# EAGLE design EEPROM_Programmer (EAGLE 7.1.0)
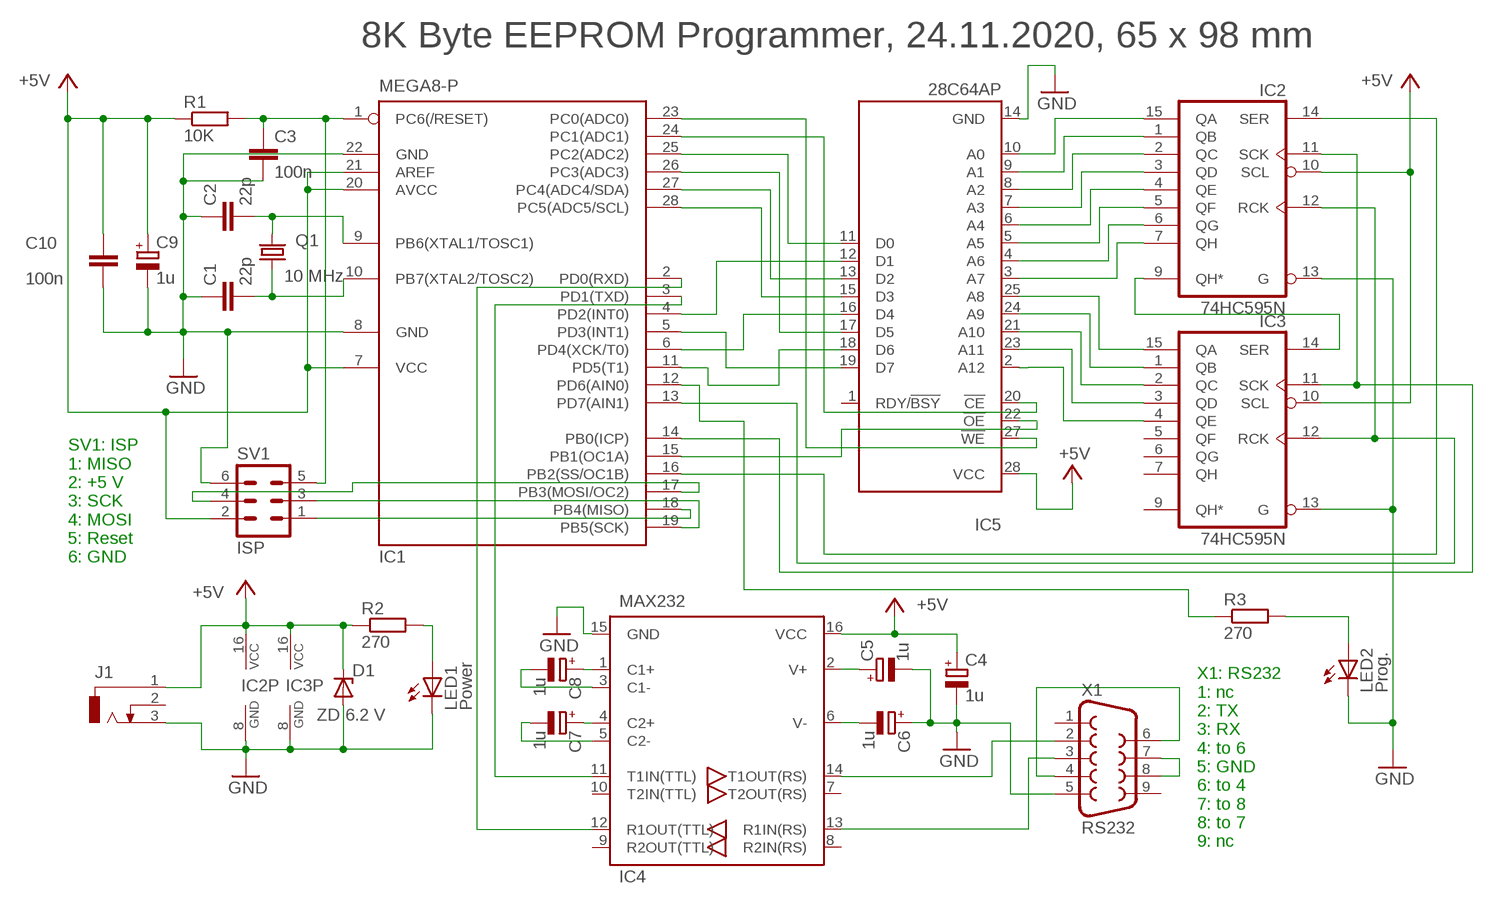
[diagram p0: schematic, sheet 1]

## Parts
C1  22p  C-EUC1206  [C1206]
C2  22p  C-EUC1206  [C1206]
C3  100n  C-EUC1206  [C1206]
C4  1u  CPOL-EUE2.5-5  [E2,5-5]
C5  1u  CPOL-EUE2.5-5  [E2,5-5]
C6  1u  CPOL-EUE2.5-5  [E2,5-5]
C7  1u  CPOL-EUE2.5-5  [E2,5-5]
C8  1u  CPOL-EUE2.5-5  [E2,5-5]
C9  1u  CPOL-EUE2.5-5  [E2,5-5]
C10  100n  C-EUC1206  [C1206]
D1  ZD 6.2 V  ZPD  [DO35Z10]
IC1  MEGA8-P  [DIL28-3]
IC2  74HC595N  [DIL16]
IC3  74HC595N  [DIL16]
IC4  MAX232-1  [DIL16]
IC5  28C64AP  [DIL28-6]
J1  DCJ0303  [DCJ0303]
LED1  Power  LED3MM  [LED3MM]
LED2  Prog.  LED3MM  [LED3MM]
Q1  10 MHz  CRYTALHC18U-V  [HC18U-V]
R1  10K  R-EU_R1206  [R1206]
R2  270  R-EU_R1206  [R1206]
R3  270  R-EU_R1206  [R1206]
SV1  ISP  ML6  [ML6]
X1  RS232  F09HP  [F09HP]

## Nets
+5V: C4.+ C9.+ C10.1 D1.C IC1.7(VCC) IC1.20(AVCC) IC1.21(AREF) IC2.10(SCL) IC2.16(VCC) IC3.10(SCL) IC3.16(VCC) IC4.16(VCC) IC5.28(VCC) J1.1 R1.1 R2.1 SV1.2
GND: C1.1 C2.1 C3.2 C4.- C5.- C6.+ C9.- C10.2 D1.A IC1.8(GND) IC1.22(GND) IC2.8(GND) IC2.13(G) IC3.8(GND) IC3.13(G) IC4.15(GND) IC5.14(GND) J1.3 LED1.K(C) LED2.K(C) SV1.6 X1.5
N$1: IC2.15(QA) IC5.10(A0)
N$2: IC2.1(QB) IC5.9(A1)
N$3: IC2.2(QC) IC5.8(A2)
N$4: IC2.3(QD) IC5.7(A3)
N$5: IC2.4(QE) IC5.6(A4)
N$6: IC2.5(QF) IC5.5(A5)
N$7: IC2.6(QG) IC5.4(A6)
N$8: IC2.7(QH) IC5.3(A7)
N$9: IC3.15(QA) IC5.25(A8)
N$10: IC3.1(QB) IC5.24(A9)
N$11: IC3.2(QC) IC5.21(A10)
N$12: IC3.3(QD) IC5.23(A11)
N$13: IC3.4(QE) IC5.2(A12)
N$14: IC2.9(QH*) IC3.14(SER)
N$15: IC1.14(PB0(ICP)) IC2.11(SCK) IC3.11(SCK)
N$16: IC1.13(PD7(AIN1)) IC2.12(RCK) IC3.12(RCK)
N$17: IC1.6(PD4(XCK/T0)) IC5.16(D4)
N$18: X1.7 X1.8
N$19: IC1.28(PC5(ADC5/SCL)) IC5.15(D3)
N$20: C2.2 IC1.9(PB6(XTAL1/TOSC1)) Q1.2
N$21: C1.2 IC1.10(PB7(XTAL2/TOSC2)) Q1.1
N$22: C3.1 IC1.1(PC6(/RESET)) R1.2 SV1.5
N$23: IC1.18(PB4(MISO)) SV1.1
N$24: IC1.2(PD0(RXD)) IC4.12(R1OUT(TTL))
N$25: C8.+ IC4.1(C1+)
N$26: C8.- IC4.3(C1-)
N$27: C6.- IC4.6(V-)
N$28: C7.+ IC4.4(C2+)
N$29: C7.- IC4.5(C2-)
N$30: C5.+ IC4.2(V+)
N$31: IC1.27(PC4(ADC4/SDA)) IC5.13(D2)
N$32: IC1.4(PD2(INT0)) IC5.12(D1)
N$33: IC1.26(PC3(ADC3)) IC5.17(D5)
N$34: IC1.25(PC2(ADC2)) IC5.11(D0)
N$35: IC1.5(PD3(INT1)) IC5.19(D7)
N$36: IC1.24(PC1(ADC1)) IC5.20(!CE)
N$37: IC1.23(PC0(ADC0)) IC5.27(!WE)
N$38: IC4.14(T1OUT(RS)) X1.2
N$39: IC1.19(PB5(SCK)) SV1.3
N$40: IC1.16(PB2(SS/OC1B)) IC2.14(SER)
N$41: IC1.17(PB3(MOSI/OC2)) SV1.4
N$42: IC4.13(R1IN(RS)) X1.3
N$43: IC1.11(PD5(T1)) IC5.18(D6)
N$44: IC1.3(PD1(TXD)) IC4.11(T1IN(TTL))
N$45: LED1.A R2.2
N$46: IC1.12(PD6(AIN0)) R3.1
N$47: LED2.A R3.2
N$48: IC1.15(PB1(OC1A)) IC5.22(!OE)
N$50: X1.4 X1.6
Unconnected: IC3.5(QF) IC3.6(QG) IC3.7(QH) IC3.9(QH*) IC4.7(T2OUT(RS)) IC4.8(R2IN(RS)) IC4.9(R2OUT(TTL)) IC4.10(T2IN(TTL)) IC5.1(RDY/!BSY) J1.2 X1.1 X1.9

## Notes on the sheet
- 8K Byte EEPROM Programmer, 24.11.2020, 65 x 98 mm
- SV1: ISP
  1: MISO
  2: +5 V
  3: SCK
  4: MOSI
  5: Reset
  6: GND
- X1: RS232
  1: nc
  2: TX
  3: RX
  4: to 6
  5: GND
  6: to 4
  7: to 8
  8: to 7
  9: nc

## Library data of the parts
C1-C3 C10 = rcl:C-EU: CAPACITOR, European symbol
C4-C9 = rcl:CPOL-EU: POLARIZED CAPACITOR, European symbol
D1 = diode:ZPD: Z DIODE
IC1 = atmel:MEGA8-P: MICROCONTROLLER 8 Kbytes FLASH, 1 kbytes SRAM, 512 bytes EEPROM, USART, 4-channel 10 bit ADC, 2-channel 8 bit ADC Pin compatible with Atmega48, ATMega88, ATMega168 Source: avr.lbr; OC_FARNELL: unknown; OC_NEWARK: unknown
IC2 IC3 = 74xx-eu:74*595: 8-bit SHIFT REGISTER, output latch
IC4 = 11manni:MAX232-1
IC5 = microchip:28*64A: CMOS EEPROM 64 K (8 K x 8), low voltage; MPN: AT28C64B-15PU; OC_FARNELL: 1631144; OC_NEWARK: 96K6557
J1 = con-jack:DCJ0303: DC POWER JACK Source: DCJ0303.pdf; OC_FARNELL: unknown; OC_NEWARK: unknown
LED1 LED2 = led:LED: LED
Q1 = 11manni:CRYTAL: CRYSTAL
R1-R3 = rcl:R-EU_: RESISTOR, European symbol
SV1 = con-harting-ml:ML6: HARTING; OC_FARNELL: unknown; OC_NEWARK: unknown
X1 = con-subd:F09: SUB-D; OC_FARNELL: unknown; OC_NEWARK: unknown

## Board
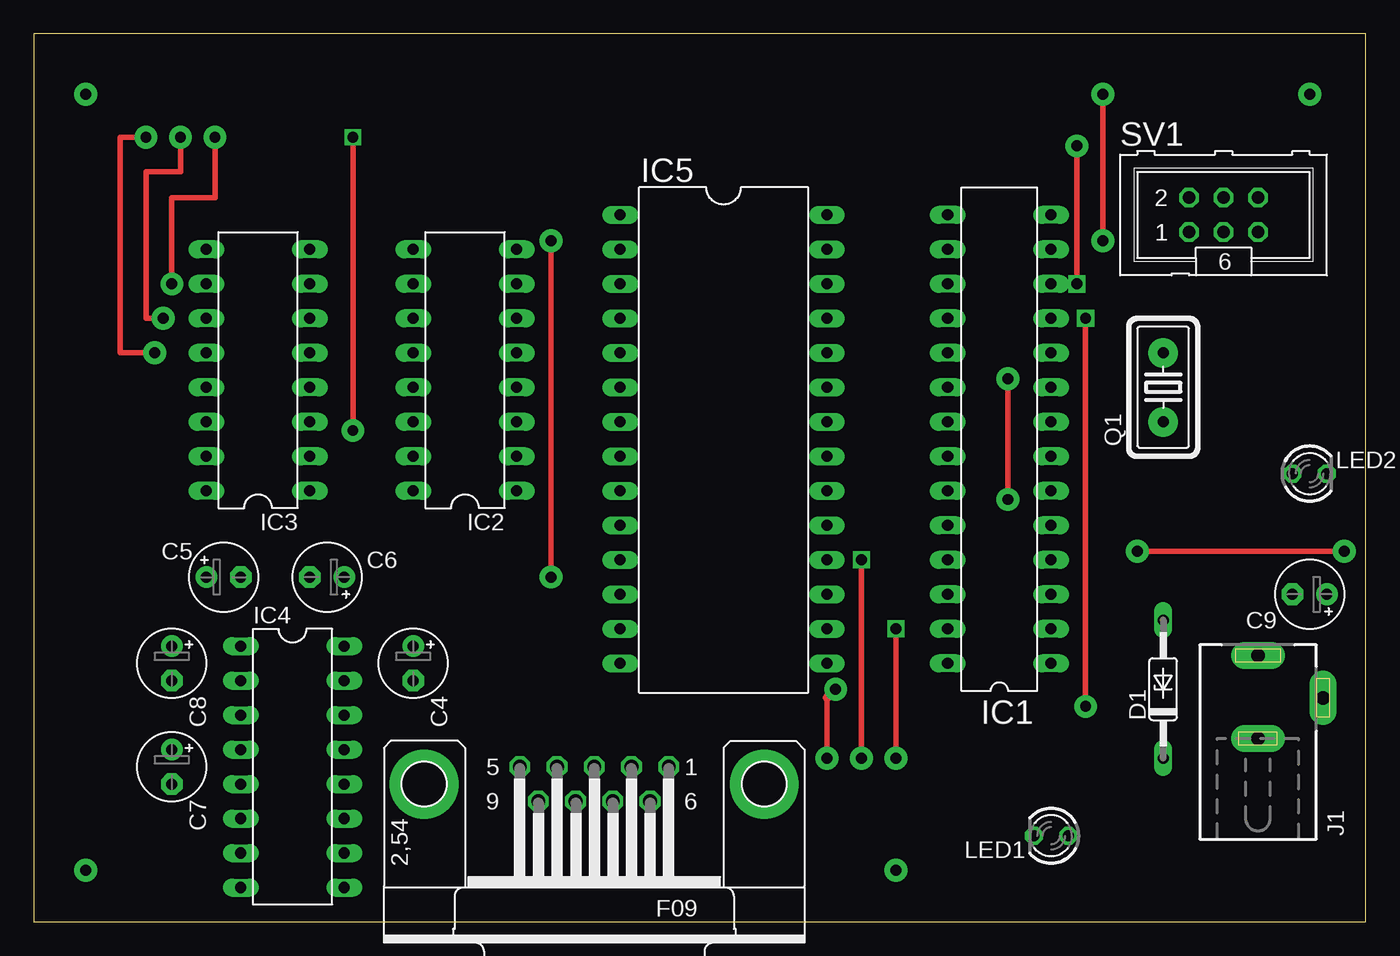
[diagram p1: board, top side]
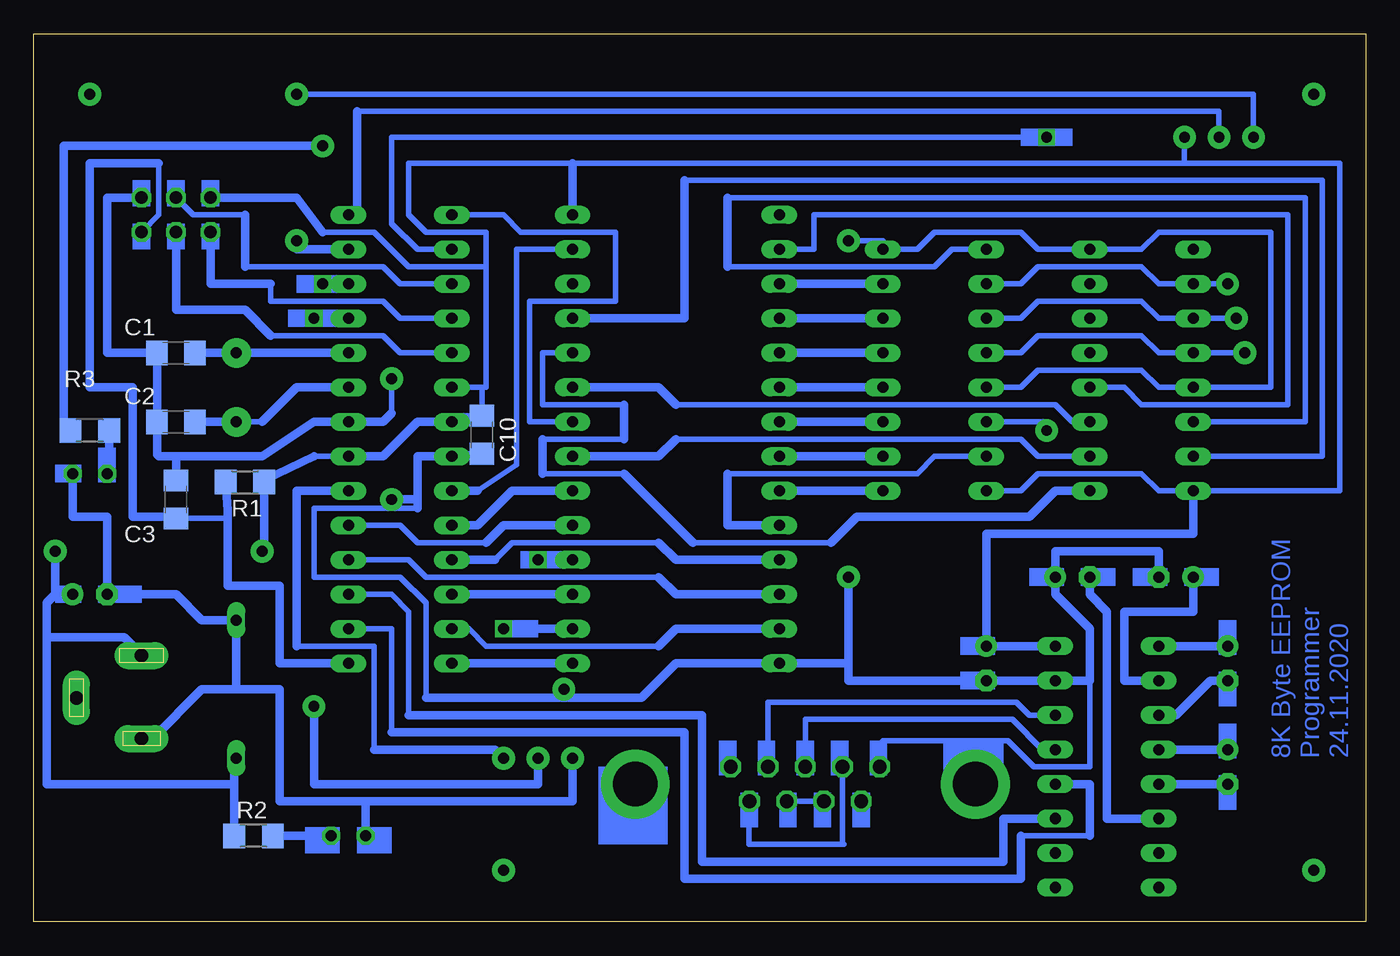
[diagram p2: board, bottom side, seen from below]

Size 98.09 x 65.39 mm. Coordinates in mm from the lower left corner, seen from the top.
Outline: 0,0 98.09,0 98.09,65.39 0,65.39 0,0
Copper layers (1*16): Top 0.035mm / dielectric 1.5mm / Bottom 0.035mm
Design rules "default": minimum track width 10mil, minimum drill 24mil, track to track 8mil, track to pad 8mil, pad to pad 8mil, via to via 8mil, smd to smd 8mil, copper to edge 40mil, drill to drill 8mil, minimum pad ring 10mil, minimum via ring 8mil, stop-mask expansion 4mil, vias tented up to drill 0mil, thermal gap 10mil

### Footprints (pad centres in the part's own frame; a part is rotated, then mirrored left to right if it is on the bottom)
C1206 = smd 1.6 x 1.8: 1 -1.4,0; 2 1.4,0
E2,5-5 = drill 0.813 pad 1.6: + -1.27,0 | drill 0.813 pad 1.6 octagon: - 1.27,0
DO35Z10 = drill 0.813 long: A 5.08,0; C -5.08,0
DIL28-3 = drill 0.813 long: 1 -16.51,-3.81; 2 -13.97,-3.81; 3 -11.43,-3.81; 4 -8.89,-3.81; 5 -6.35,-3.81; 6 -3.81,-3.81; 7 -1.27,-3.81; 8 1.27,-3.81; 9 3.81,-3.81; 10 6.35,-3.81; 11 8.89,-3.81; 12 11.43,-3.81; 13 13.97,-3.81; 14 16.51,-3.81; 15 16.51,3.81; 16 13.97,3.81; 17 11.43,3.81; 18 8.89,3.81; 19 6.35,3.81; 20 3.81,3.81; 21 1.27,3.81; 22 -1.27,3.81; 23 -3.81,3.81; 24 -6.35,3.81; 25 -8.89,3.81; 26 -11.43,3.81; 27 -13.97,3.81; 28 -16.51,3.81
DIL16 = drill 0.813 long: 1 -8.89,-3.81; 2 -6.35,-3.81; 3 -3.81,-3.81; 4 -1.27,-3.81; 5 1.27,-3.81; 6 3.81,-3.81; 7 6.35,-3.81; 8 8.89,-3.81; 9 8.89,3.81; 10 6.35,3.81; 11 3.81,3.81; 12 1.27,3.81; 13 -1.27,3.81; 14 -3.81,3.81; 15 -6.35,3.81; 16 -8.89,3.81
DIL28-6 = drill 0.813 long: 1 -16.51,-7.62; 2 -13.97,-7.62; 3 -11.43,-7.62; 4 -8.89,-7.62; 5 -6.35,-7.62; 6 -3.81,-7.62; 7 -1.27,-7.62; 8 1.27,-7.62; 9 3.81,-7.62; 10 6.35,-7.62; 11 8.89,-7.62; 12 11.43,-7.62; 13 13.97,-7.62; 14 16.51,-7.62; 15 16.51,7.62; 16 13.97,7.62; 17 11.43,7.62; 18 8.89,7.62; 19 6.35,7.62; 20 3.81,7.62; 21 1.27,7.62; 22 -1.27,7.62; 23 -3.81,7.62; 24 -6.35,7.62; 25 -8.89,7.62; 26 -11.43,7.62; 27 -13.97,7.62; 28 -16.51,7.62
DCJ0303 = drill 1 pad 2 long: 1 0,3.1; 2 4.8,0; 3 0,-3
LED3MM = drill 0.813 octagon: A -1.27,0; K 1.27,0
HC18U-V = drill 0.813 pad 2.184: 1 -2.54,0; 2 2.54,0
R1206 = smd 1.6 x 1.803: 1 -1.422,0; 2 1.422,0
ML6 = drill 0.914 octagon: 1 -2.54,-1.27; 2 -2.54,1.27; 3 0,-1.27; 4 0,1.27; 5 2.54,-1.27; 6 2.54,1.27
F09HP = drill 1.016 octagon: 1 -5.486,-1.27; 2 -2.743,-1.27; 3 0,-1.27; 4 2.743,-1.27; 5 5.486,-1.27; 6 -4.115,1.27; 7 -1.372,1.27; 8 1.372,1.27; 9 4.115,1.27 | drill 3.302 pad 5.08: G1 -12.522,0; G2 12.522,0

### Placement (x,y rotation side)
C1  87.63,41.91 0 bottom
C2  87.63,36.83 0 bottom
C3  87.63,31.11 90 bottom
C4  27.94,19.05 270 top
C5  13.97,25.4 0 top
C6  21.59,25.4 180 top
C7  10.16,11.43 270 top
C8  10.16,19.05 270 top
C9  93.98,24.13 180 top
C10  65.09,35.88 270 bottom
D1  83.19,17.14 90 top
IC1  71.12,35.56 90 top
IC2  31.75,40.64 90 top
IC3  16.51,40.64 90 top
IC4  19.05,11.43 270 top
IC5  50.8,35.56 270 top
J1  90.17,16.51 0 top
LED1  74.93,6.35 180 top
LED2  93.98,33.02 0 top
Q1  83.19,39.37 270 top
R1  82.55,32.38 180 bottom
R2  81.92,6.35 0 bottom
R3  93.98,36.2 0 bottom
SV1  87.63,52.07 0 top
X1  41.27,10.16 180 top

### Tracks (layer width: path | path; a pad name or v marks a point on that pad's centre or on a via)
+5V  (via drill 0.8 pad 1.68)
  Top 0.406: v81.28,27.3 v96.52,27.3 | v10.16,46.99 10.16,53.34 13.34,53.34 v13.34,57.78
  Bottom 0.406: IC2.16 25.4,31.75 24.13,33.02 16.51,33.02 15.24,31.75 IC3.16 1.91,31.75 1.91,55.88 13.34,55.88 | R1.1 81.13,32.54 | 77.47,34.29 IC1.7 | IC1.20 65.09,39.37 | 65.09,39.37 64.77,39.37 64.77,48.26 | 13.34,55.88 58.42,55.88 70.48,55.88 70.48,52.07 69.22,50.8 64.77,50.8 64.77,48.26 | 76.83,50.8 73.03,50.8 70.48,48.26 64.77,48.26 | 65.09,39.37 C10.1 67.31,37.28 IC1.21 | IC2.10 25.4,46.99 24.13,48.26 16.51,48.26 15.24,46.99 IC3.10 v10.16,46.99 | v13.34,57.78 13.34,55.88
  Bottom 0.61: 81.13,32.54 77.47,34.29 | IC1.7 72.39,34.29 69.85,36.83 IC1.21 | IC4.16 C4.+ 27.94,28.57 12.7,28.57 IC3.16 | IC5.28 58.42,55.88 | SV1.2 78.74,53.34 76.83,50.8 | R1.1 81.13,27.46 v81.28,27.3 | v96.52,27.3 96.52,24.13 | R2.1 83.34,10.16 | 83.34,10.16 83.34,11.91 D1.C | C9.+ 96.52,24.13 | 83.34,10.16 97.16,10.16 97.16,20.95 | 97.16,20.95 97.16,23.5 96.52,24.13 | J1.1 90.09,19.61 91.44,20.95 97.16,20.95
GND  (via drill 0.8 pad 1.68)
  Top 0.406: v38.1,25.4 v38.1,50.16 | v71.75,40.01 v71.75,31.11 | v58.42,12.06 58.42,16.51
  Top 0.61: 58.42,16.51 v59.05,17.14
  Bottom 0.406: 89.03,34.42 88.9,34.29 | 69.85,30.48 77.47,30.48 77.47,25.4 71.12,25.4 69.22,23.5 69.22,16.51 | v38.1,50.16 35.56,50.16 IC2.8 33.02,49.53 31.75,50.8 25.4,50.8 24.13,49.53 IC3.8 16.51,49.53 15.24,50.8 6.99,50.8 6.99,39.37 IC3.13 15.24,39.37 16.51,40.64 24.13,40.64 25.4,39.37 IC2.13 | 71.75,37.47 v71.75,40.01 | C10.2 67.31,34.48 IC1.22 | X1.5 35.79,13.11 35.56,13.34 26.35,13.34 24.45,11.43 20.32,11.43 20.32,17.78
  Bottom 0.61: 89.03,34.42 C2.1 C1.1 92.71,41.91 92.71,53.34 SV1.6 | 88.9,34.29 87.63,34.29 | 87.63,34.29 81.28,34.29 77.47,36.83 IC1.8 72.39,36.83 71.75,37.47 | C3.2 87.63,34.29 | IC1.22 69.85,34.29 69.85,31.11 | 69.85,31.11 69.85,30.48 | 69.22,16.51 59.05,16.51 | 59.05,16.51 53.34,16.51 50.8,19.05 IC5.14 38.1,19.05 | 38.1,19.05 v38.1,25.4 | C5.- 15.24,27.3 22.86,27.3 C6.+ 22.86,24.13 20.32,21.59 20.32,17.78 IC4.15 C4.- 38.1,17.78 38.1,19.05 | v71.75,31.11 69.85,31.11 | v59.05,17.14 59.05,16.51 | v58.42,12.06 58.42,8.89 73.66,8.89 | 73.66,8.89 80.01,8.89 80.01,17.14 83.19,17.14 | 83.19,17.14 D1.A 85.72,22.23 87.63,24.13 C9.- 92.71,29.84 95.25,29.84 LED2.K | LED1.K 73.66,8.89 | J1.3 89.36,13.51 85.72,17.14 83.19,17.14
N$1
  Bottom 0.406: IC2.15 31.75,34.29 33.02,33.02 46.99,33.02
  Bottom 0.61: 46.99,33.02 46.99,29.21 IC5.10
N$2
  Bottom 0.61: IC2.1 IC5.9
N$3
  Bottom 0.61: IC2.2 IC5.8
N$4
  Bottom 0.61: IC2.3 IC5.7
N$5
  Bottom 0.61: IC2.4 IC5.6
N$6
  Bottom 0.61: IC2.5 IC5.5
N$7
  Bottom 0.61: IC2.6 IC5.4
N$8
  Bottom 0.61: IC2.7 IC5.3
N$9
  Bottom 0.406: IC3.15 3.17,34.29 3.17,54.61 50.16,54.61
  Bottom 0.61: 50.16,54.61 50.16,44.45 IC5.25
N$10
  Bottom 0.406: 39.37,27.94 49.53,27.94 | 54.61,33.02 60.64,33.02 | 60.64,35.56 54.61,35.56 | 54.61,38.1 60.64,38.1 60.64,41.91 IC5.24
  Bottom 0.61: IC3.1 22.86,31.75 24.77,29.84 37.47,29.84 39.37,27.94 | 49.53,27.94 54.61,33.02 | 60.64,33.02 60.64,35.56 | 54.61,35.56 54.61,38.1
N$11
  Bottom 0.406: IC3.2 24.13,34.29 25.4,35.56 50.8,35.56
  Bottom 0.61: 50.8,35.56 52.07,34.29 IC5.21
N$12
  Bottom 0.406: IC3.3 21.59,36.83 22.86,38.1 50.8,38.1
  Bottom 0.61: 50.8,38.1 52.07,39.37 IC5.23
N$13
  Bottom 0.406: IC3.4 17.78,39.37 16.51,38.1 5.71,38.1 5.71,52.07 40.64,52.07 40.64,49.53 IC5.2
N$14
  Bottom 0.406: IC3.14 4.45,36.83 4.45,53.34 46.99,53.34 | 46.99,48.26 31.75,48.26 30.48,49.53 IC2.9
  Bottom 0.61: 46.99,53.34 46.99,48.26
N$15  (via drill 0.8 pad 1.68)
  Top 0.406: v10.79,57.78 10.79,55.24 8.26,55.24 8.26,44.45 v9.53,44.45
  Bottom 0.406: IC2.11 25.4,44.45 24.13,45.72 16.51,45.72 15.24,44.45 IC3.11 v9.53,44.45 | 74.3,59.69 10.79,59.69 v10.79,57.78
  Bottom 0.61: IC1.14 74.3,52.07 74.3,59.69
N$16  (via drill 0.8 pad 1.68)
  Top 0.406: v8.26,57.78 6.35,57.78 6.35,41.91 v8.89,41.91 | v78.74,50.16 v78.74,60.96
  Bottom 0.406: IC2.12 25.4,41.91 24.13,43.18 16.51,43.18 15.24,41.91 IC3.12 v8.89,41.91 | v78.74,60.96 8.26,60.96 v8.26,57.78
  Bottom 0.61: IC1.13 78.74,49.53 v78.74,50.16
N$17  (via drill 0.8 pad 1.27, 0.8 pad 1.68)
  Top 0.406: v63.5,21.59 v63.5,12.06
  Bottom 0.406: 78.74,20.32 73.03,20.32 73.03,12.7
  Bottom 0.61: IC5.16 v63.5,21.59 | IC1.6 78.74,31.75 78.74,20.32 | 73.03,12.7 64.14,12.7 v63.5,12.06
N$18
  Bottom 0.406: X1.7 X1.8
N$19
  Bottom 0.61: IC1.28 IC5.15
N$20
  Bottom 0.406: 81.28,36.83 Q1.2
  Bottom 0.61: IC1.9 78.74,39.37 81.28,36.83 | C2.2 Q1.2
N$21
  Bottom 0.61: IC1.10 Q1.1 C1.2
N$22
  Bottom 0.406: 83.82,24.77 83.95,29.71 C3.1 87.76,29.84 | SV1.5 88.9,52.07 88.9,55.88
  Bottom 0.61: R1.2 83.82,30.33 83.82,24.77 80.01,24.77 80.01,19.05 IC1.1 | 88.9,55.88 93.98,55.88 93.98,39.37 90.81,39.37 90.81,29.84 87.76,29.84
N$23
  Bottom 0.406: 80.64,46.99 80.64,45.72 72.39,45.72 71.12,44.45 IC1.18
  Bottom 0.61: SV1.1 85.09,46.99 80.64,46.99
N$24
  Bottom 0.406: IC1.2 71.75,21.59 71.75,13.97 | 25.4,6.35 20.32,6.35
  Bottom 0.61: 71.75,13.97 50.16,13.97 50.16,3.17 25.4,3.17 25.4,6.35 | 20.32,6.35 20.32,10.16 IC4.12
N$25
  Bottom 0.61: IC4.1 C8.+
N$26
  Bottom 0.406: IC4.3 13.97,15.24
  Bottom 0.61: 13.97,15.24 11.43,17.78 C8.-
N$27
  Bottom 0.61: C6.- 20.32,24.13 19.05,22.86 19.05,7.62 IC4.6
N$28
  Bottom 0.61: IC4.4 C7.+
N$29
  Bottom 0.61: IC4.5 C7.-
N$30
  Bottom 0.61: IC4.2 17.78,17.78 17.78,22.86 12.7,22.86 C5.+
N$31
  Bottom 0.406: IC1.27 66.04,21.59 64.77,20.32 52.07,20.32
  Bottom 0.61: 52.07,20.32 50.8,21.59 IC5.13
N$32
  Bottom 0.406: IC1.4 70.48,26.67 69.22,25.4 52.07,25.4
  Bottom 0.61: 52.07,25.4 50.8,24.13 IC5.12
N$33
  Bottom 0.61: IC1.26 IC5.17
N$34
  Bottom 0.406: 64.14,26.67 62.87,27.94 52.07,27.94
  Bottom 0.61: IC1.25 64.14,26.67 | 52.07,27.94 50.8,26.67 IC5.11
N$35
  Bottom 0.406: IC1.5 71.12,29.21 69.85,27.94 64.77,27.94
  Bottom 0.61: 64.77,27.94 63.5,29.21 IC5.19
N$36
  Bottom 0.61: IC1.24 65.41,29.21 62.87,31.75 IC5.20
N$37
  Bottom 0.406: 65.41,31.75 62.55,33.66 62.55,49.53 IC5.27
  Bottom 0.61: IC1.23 65.41,31.75
N$38
  Bottom 0.406: IC4.14 24.77,15.24 25.72,16.19 44.02,16.19 X1.2
N$39
  Bottom 0.406: 80.64,43.18 72.39,43.18 71.12,41.91 IC1.19
  Bottom 0.61: SV1.3 87.63,45.09 82.55,45.09 80.64,43.18
N$40  (via drill 0.8 pad 1.02, 0.8 pad 1.68)
  Top 0.406: v23.5,57.78 v23.5,36.2
  Bottom 0.406: IC2.14 23.5,36.83 v23.5,36.2 | IC1.16 69.85,49.53 71.75,51.44 71.75,57.78 v23.5,57.78
N$41
  Bottom 0.406: SV1.4 86.36,52.07 82.55,52.07 | 82.55,48.26 72.39,48.26 71.12,46.99 IC1.17
  Bottom 0.61: 82.55,52.07 82.55,48.26
N$42
  Bottom 0.406: IC4.13 23.81,12.7 26.04,14.92 41.27,14.92 X1.3
N$43  (via drill 0.8 pad 1.27, 0.8 pad 1.68)
  Top 0.406: v77.47,44.45 v77.47,15.88 | v60.96,26.67 v60.96,12.06
  Bottom 0.406: IC5.18 v60.96,26.67 | IC1.11 v77.47,44.45
  Bottom 0.61: v77.47,15.88 77.47,10.16 60.96,10.16 v60.96,12.06
N$44
  Bottom 0.406: IC1.3 71.75,24.13 70.48,22.86 70.48,15.24
  Bottom 0.61: 70.48,15.24 48.9,15.24 48.9,4.45 26.67,4.45 26.67,7.62 IC4.11
N$45
  Bottom 0.61: LED1.A R2.2
N$46  (via drill 0.8 pad 1.27, 0.8 pad 1.68)
  Top 0.406: v76.83,57.15 v76.83,46.99
  Bottom 0.61: v76.83,57.15 95.89,57.15 95.89,36.68 R3.1 | v76.83,46.99 IC1.12
N$47
  Bottom 0.61: R3.2 92.56,33.17 LED2.A
N$48
  Bottom 0.406: IC5.22 61.59,36.83 61.59,45.72 55.24,45.72 55.24,50.8 62.23,50.8 63.5,52.07 IC1.15
N$49  (via drill 0.8 pad 1.68)
  other vias: 3.81,60.96
N$50
  Bottom 0.406: X1.6 45.4,8.89 45.4,5.71 38.53,5.71 | 38.42,5.71 38.53,5.71 | 38.53,5.71 X1.4
N$51  (via drill 0.8 pad 1.68)
  other vias: 93.98,60.96
N$52  (via drill 0.8 pad 1.68)
  other vias: 63.5,3.81
N$53  (via drill 0.8 pad 1.68)
  other vias: 3.81,3.81
(copper drawn outside any net)
  shapes: Bottom area x40

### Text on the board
Bottom: 8K Byte EEPROM / Programmer / 24.11.2020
